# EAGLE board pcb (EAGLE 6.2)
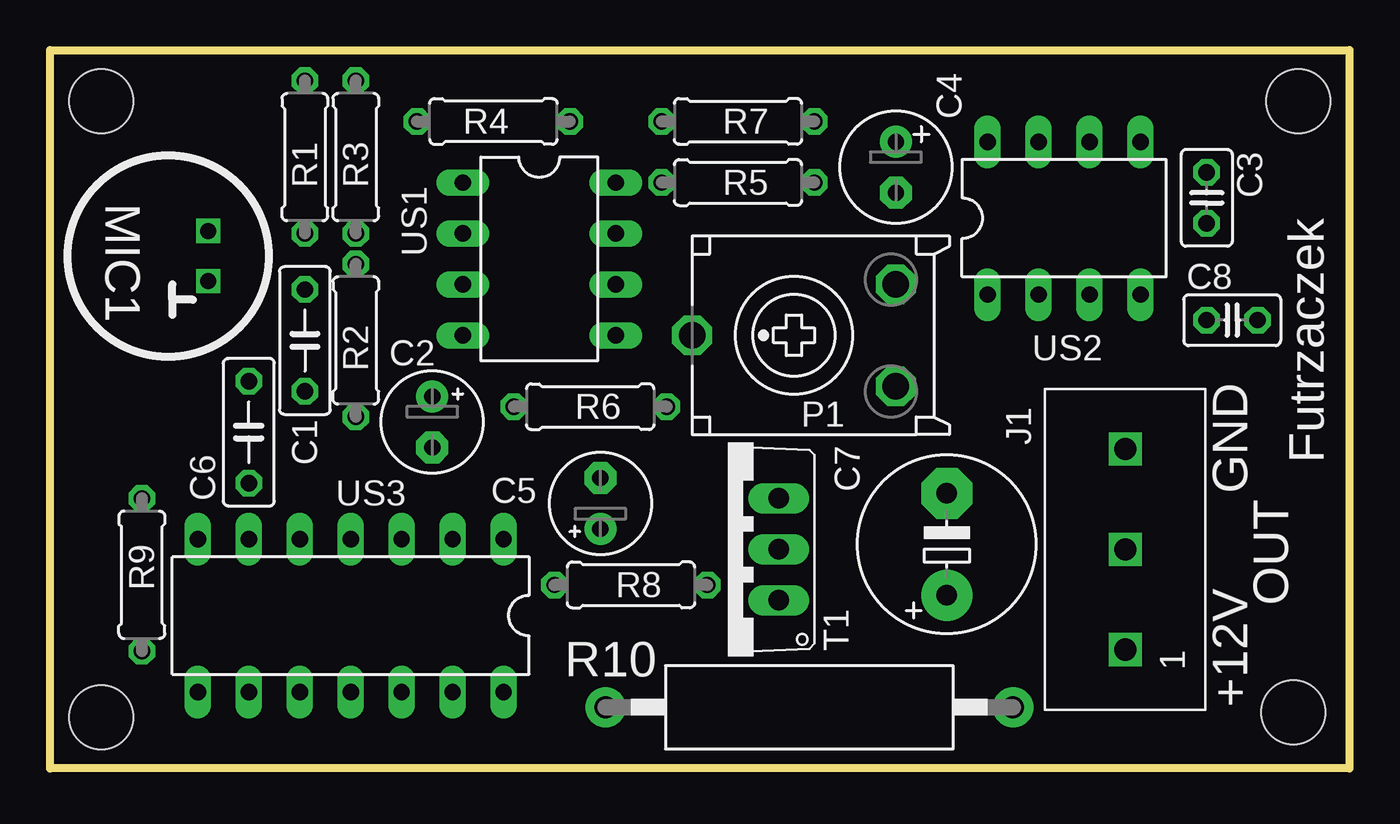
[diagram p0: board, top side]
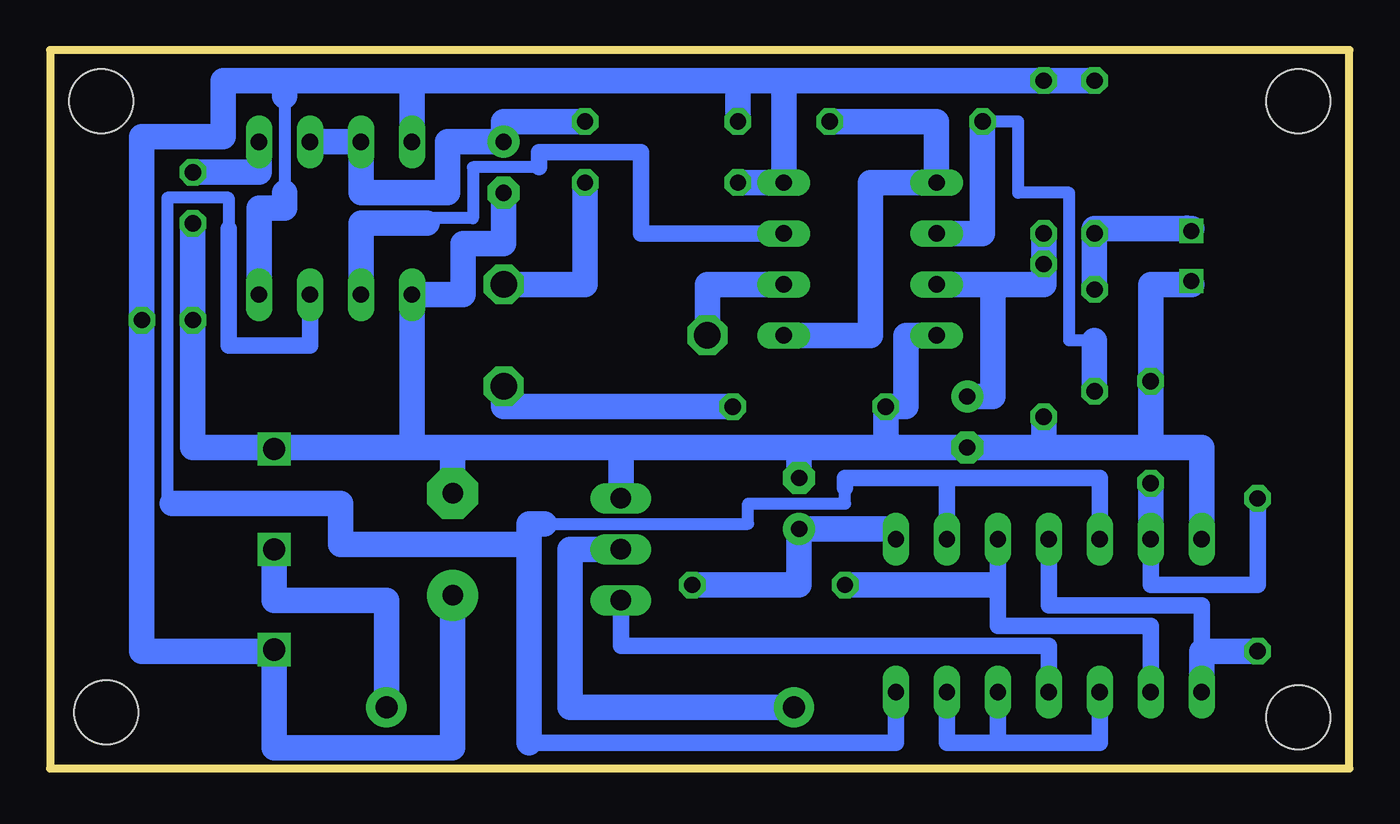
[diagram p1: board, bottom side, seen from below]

Size 64.77 x 35.81 mm. Coordinates in mm from the lower left corner, seen from the top.
Outline: 0,35.81 64.77,35.81 64.77,0 0,0 0,35.81
Copper layers (1*16): Top 0.035mm / dielectric 1.5mm / Bottom 0.035mm
Design rules: minimum track width 10mil, minimum drill 24mil, track to track 8mil, track to pad 8mil, pad to pad 8mil, via to via 8mil, smd to smd 8mil, copper to edge 40mil, drill to drill 8mil, minimum pad ring 10mil, minimum via ring 8mil, stop-mask expansion 4mil, vias tented up to drill 0mil, thermal gap 10mil
Holes 3.2 mm at 2.54,33.27 2.54,2.54 61.98,2.79 62.23,33.27

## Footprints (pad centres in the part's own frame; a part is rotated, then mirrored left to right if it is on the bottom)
C050-025X075 = drill 0.813 octagon: 1 -2.54,0; 2 2.54,0
E2,5-5 = drill 0.813 pad 1.6: + -1.27,0 | drill 0.813 pad 1.6 octagon: - 1.27,0
C025-025X050 = drill 0.813 octagon: 1 -1.27,0; 2 1.27,0
E2,5-6 = drill 0.813 pad 1.6: + -1.27,0 | drill 0.813 pad 1.6 octagon: - 1.27,0
E5-8,5 = drill 1.016 pad 2.54: + -2.54,0 | drill 1.016 pad 2.54 octagon: - 2.54,0
3PIN-5MM = drill 1.1 square: P$1 -5,0; P$2 0,0; P$3 5,0
ECP10S = drill 1.321 octagon: A -2.54,-5.08; E 2.54,-5.08; S 0,5.08
0207/7 = drill 0.813 octagon: 1 -3.81,0; 2 3.81,0
CA0002 = drill 1.1 pad 2: 1 -10.16,0; 2 10.16,0
TO220V = drill 1.016 long: 1 -2.54,-2.54; 2 0,-2.54; 3 2.54,-2.54
DIL08 = drill 0.813 long: 1 -3.81,-3.81; 2 -1.27,-3.81; 3 1.27,-3.81; 4 3.81,-3.81; 5 3.81,3.81; 6 1.27,3.81; 7 -1.27,3.81; 8 -3.81,3.81
DIL14 = drill 0.813 long: 1 -7.62,-3.81; 2 -5.08,-3.81; 3 -2.54,-3.81; 4 0,-3.81; 5 2.54,-3.81; 6 5.08,-3.81; 7 7.62,-3.81; 8 7.62,3.81; 9 5.08,3.81; 10 2.54,3.81; 11 0,3.81; 12 -2.54,3.81; 13 -5.08,3.81; 14 -7.62,3.81

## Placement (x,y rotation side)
C1  [C050-025X075]  12.7,21.34 90 top
C2  [E2,5-5]  19.05,17.27 270 top
C3  [C025-025X050]  57.66,28.45 270 top
C4  [E2,5-6]  42.16,29.97 270 top
C5  [E2,5-5]  27.43,13.21 90 top
C6  [C050-025X075]  9.91,16.76 90 top
C7  [E5-8,5]  44.7,11.18 90 top
C8  [C025-025X050]  58.93,22.35 0 top
J1  [3PIN-5MM]  53.59,10.92 90 top
P1  [ECP10S]  37.08,21.59 90 top
R1  [0207/7]  12.7,30.48 90 top
R2  [0207/7]  15.24,21.34 90 top
R3  [0207/7]  15.24,30.48 90 top
R4  [0207/7]  22.1,32.26 0 top
R5  [0207/7]  34.29,29.21 180 top
R6  [0207/7]  26.92,18.03 180 top
R7  [0207/7]  34.29,32.26 180 top
R8  [0207/7]  28.96,9.14 180 top
R9  [0207/7]  4.57,9.65 270 top
R10  [CA0002]  37.85,3.05 0 top
T1  [TO220V]  33.78,10.92 90 top
US1  [DIL08]  24.38,25.4 270 top
US2  [DIL08]  50.55,27.43 0 top
US3  [DIL14]  14.99,7.62 180 top

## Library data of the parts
C1-C8 R1-R9 = rcl
J1 = zlacza_futrzak
P1 = pot
R10 = resistor-power
T1 = transistor-npn
US1-US3 = 40xx

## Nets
S$3: R4.2 US1.1 US1.5
S$4: C4.-
S$5: US1.7
S$6: C3.1
S$7: C2.+ R3.1
S$8: P1.S US1.6
S$9: J1.P$2 R10.2
S$10: R1.1
S$11: R4.1 US1.2
S$13: P1.A R6.1
S$14: US1.4
S$15: C3.2 C5.- C7.- R2.1 R6.2
S$16: C4.+ R7.1 US2.6 US2.7
S$17: P1.E R5.1
S$21: US2.2
S$22: US3.14
S$23: US2.4
S$30: C7.+ R1.2 R3.2 R7.2
S$31: US2.3 US3.2 US3.5
S$32: US3.3 US3.9
S$33: R8.2
S$34: R9.1 US3.6
S$36: C5.+ R8.1 US3.1
S$37: R9.2 US3.4
S$38: T1.3
S$39: US3.10 US3.12 US3.13
S$40: T1.1 US3.11
S$41: T1.2

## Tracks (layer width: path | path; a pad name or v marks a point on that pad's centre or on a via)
S$1  (via drill 0.8)
  other vias: 7.88,26.8
S$2  (via drill 0.8)
  other vias: 7.88,24.3
S$3
  Bottom 1.27: R4.2 20.57,32.26 US1.1 23.88,29.21 23.88,21.59 US1.5
S$4
  Bottom 1.27: 46.74,24.13 46.74,23.62 | 46.74,23.62 46.74,16.51 | 46.74,23.62 44.2,23.62 44.2,26.16 42.16,26.16 C4.-
S$5
  Bottom 0.61: 40.39,29.97 43.69,29.97 43.69,27.43 46.23,27.43
  Bottom 0.813: US1.7 35.31,26.67 35.31,30.73 40.39,30.73 40.39,29.97
S$6
  Bottom 1.27: C3.1 54.36,29.72 54.36,30.99
S$7
  Bottom 1.27: R3.1 15.24,24.13 17.78,24.13 | 17.78,24.13 20.83,24.13 | C2.+ 17.78,18.54 17.78,24.13
S$8
  Bottom 1.27: US1.6 32,24.13 P1.S
S$9
  Bottom 1.27: R10.2 48.01,8.38 53.59,8.38 J1.P$2
S$10
  Bottom 1.27: R1.1 12.7,23.88
S$11
  Bottom 0.61: 12.7,21.34 13.97,21.34 13.97,28.7 16.51,28.7 16.51,32.26 R4.1
  Bottom 1.27: 12.7,21.34 12.7,18.8 | R4.1 18.29,26.67 US1.2
S$12
  Bottom 1.27: 8.09,26.94 7.84,26.92 12.7,26.92
S$13
  Bottom 1.27: P1.A 42.16,18.03 R6.1
S$14
  Bottom 1.27: 22.86,18.03 22.1,18.03 22.1,21.59 US1.4
S$15
  Bottom 1.27: 7.84,24.12 9.91,24.12 9.91,16 | R6.2 23.11,16 | 23.11,16 15.24,16 | 15.24,16 R2.1 | 44.7,16 57.66,16 C3.2 | 44.7,16 27.43,16 | 27.43,16 23.11,16 | 9.91,16 15.24,16 | 7.37,10.92 7.37,16 9.91,16 | C5.- 27.43,16 | C7.- 44.7,16
S$16
  Bottom 1.27: US2.6 US2.7 49.28,28.7 44.96,28.7 44.96,31.24 C4.+ 42.16,32.26 R7.1
S$17
  Bottom 1.27: R5.1 38.1,24.13 P1.E
S$21
  Bottom 1.27: US2.2 49.28,27.18 45.97,27.18
S$22
  Bottom 0.813: 40.64,1.27 22.61,1.27 US3.14
S$23
  Bottom 1.27: US2.4 54.36,27.94 53.09,27.94 53.09,28.7
S$24
  Bottom 0.61: 53.09,33.27 53.09,28.7
S$30
  Bottom 1.27: 28.19,34.29 28.19,29.21 30.48,29.21 | 28.19,34.29 R3.2 R1.2 | 28.19,34.29 30.48,34.29 | 30.48,34.29 46.74,34.29 | 46.74,34.29 46.74,30.73 | R7.2 30.48,34.29 | 46.74,34.29 53.09,34.29 | 53.09,34.29 53.09,33.53 | 53.09,34.29 56.13,34.29 56.13,31.5 60.2,31.5 60.2,5.84 53.59,5.84 53.59,1.02 44.7,1.02 C7.+
S$31
  Bottom 0.61: 40.13,12.19 29.97,12.19 29.97,13.21 25.15,13.21 25.15,13.97 | 58.67,13.21 58.93,13.21 58.93,28.45 55.88,28.45 55.88,26.92
  Bottom 0.813: US3.5 12.45,14.48 20.07,14.48 | 20.07,14.48 US3.2 | 20.07,14.48 25.15,14.48 25.15,13.97 | US2.3 51.82,21.08 55.88,21.08 55.88,26.92
  Bottom 1.27: 40.13,12.19 40.89,12.19 40.89,11.18 | 40.89,11.18 50.29,11.18 50.29,13.21 58.67,13.21 | 40.89,11.18 40.89,1.27
S$32
  Bottom 0.813: US3.3 17.53,7.11 9.91,7.11 US3.9
S$33
  Bottom 1.27: 17.78,9.14 R8.2
S$34
  Bottom 0.813: R9.1 4.57,9.14 9.91,9.14 US3.6
  Bottom 1.27: 9.91,13.97 US3.6
S$36
  Bottom 1.27: US3.1 22.61,11.94 C5.+ 27.43,9.14 R8.1
S$37
  Bottom 0.813: US3.4 14.99,8.13 7.37,8.13 7.37,5.84
  Bottom 1.27: 7.37,3.3 7.37,5.84 R9.2
S$38
  Bottom 1.27: T1.3 36.32,15.75
S$39
  Bottom 0.813: US3.10 12.45,1.27 17.53,1.27 | 17.53,1.27 US3.12 | 17.53,1.27 20.07,1.27 US3.13
S$40
  Bottom 0.813: US3.11 14.99,6.1 36.32,6.1 T1.1
S$41
  Bottom 1.27: T1.2 38.86,10.92 38.86,3.05 27.69,3.05

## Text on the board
tNames: MIC1 | Futrzaczek | GND | OUT | +12V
